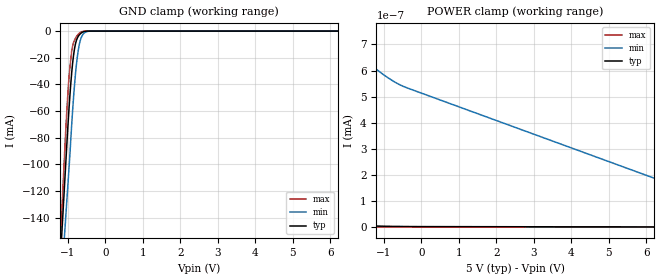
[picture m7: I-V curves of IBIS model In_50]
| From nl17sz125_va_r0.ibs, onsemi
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|//////////////////////////////////////////////////////////////////////////////
|//////////////////////////////////////////////////////////////////////////////
[Model]  In_50
Model_type Input
Vinh = 3.50
Vinl = 1.50
|  variable   typ   min   max
C_comp   2.6pF   2.6pF   2.6pF
|//////////////////////////////////////////////////////////////////////////////
[Temperature Range]   25   125   -55
|//////////////////////////////////////////////////////////////////////////////
[Voltage Range]   5.00V   4.50V   5.50V
|//////////////////////////////////////////////////////////////////////////////
[POWER Clamp Reference] 5.00V   4.50V   5.50V
|//////////////////////////////////////////////////////////////////////////////
[GND Clamp Reference]   0V   0V   0V
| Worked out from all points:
|   GND clamp passes 1 mA (typ) near -0.62 V on its own axis
|//////////////////////////////////////////////////////////////////////////////
[GND Clamp]
|   Voltage   I(typ)   I(min)   I(max)
-5V       -2.068A    -1.798A    -2.352A
-1.2V     -170.1mA   -198.9mA   -155.9mA
-1.15V    -145.1mA   -177.9mA   -127mA
-1.1V     -120.1mA   -156.9mA   -98.13mA
-1.075V   -107.7mA   -146.3mA   -83.68mA
-1V       -70.81mA   -114.8mA   -45.96mA
-900mV    -31.24mA   -70.23mA   -14.99mA
-850mV    -17.99mA   -49.56mA   -8.629mA
-775mV    -7.06mA    -25.4mA    -4.236mA
-700mV    -2.943mA   -10.43mA   -1.711mA
-625mV    -1.05mA    -3.608mA   -399.6uA
10V       2.643pA    802.3pA    833.8fA
|//////////////////////////////////////////////////////////////////////////////
[POWER Clamp]
|   Voltage   I(typ)   I(min)   I(max)
-5V       928.9uA    2.88nA     26.09mA
-4.175V   766pA      1.612nA    2.309mA
-3.95V    455.6pA    1.432nA    49.47uA
-3.725V   274.8pA    1.286nA    6.7nA
-3.65V    233pA      1.243nA    60.09pA
-3.575V   197.8pA    1.203nA    16.48pA
-3.275V   104.8pA    1.066nA    8.127pA
-2.975V   57.19pA    957.4pA    3.911pA
-2.15V    13.2pA     748.7pA    840.4fA
-1.925V   9.338pA    707.4pA    672.9fA
-500mV    2.043pA    540.5pA    554.8fA
10V       -549.2fA   -11.74pA   -177.6fA
